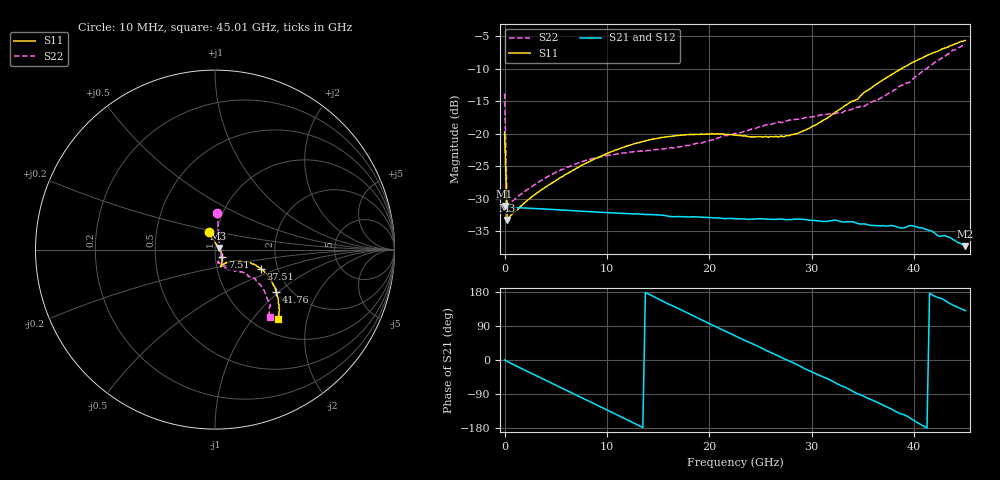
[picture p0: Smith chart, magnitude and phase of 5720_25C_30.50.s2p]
! Device:  ADRF5720
! Description: 0.5dB LSB GaAs MMIC 6-bit Digital Attenuator
! Frequency:  0.000009 -  40 GHz
! Ports:
!	RF1	= Port 1
!	RF2	= Port 2
! Vdd:  3.3 Volt
! Vss:  -3.3 Volt
! Control:  0/3.3 Volt
! State:  30.50 dB attenuation
! Data:  The device was measured using G-S-G Probes on a matrix board.
!  Data was collected using an calibrated 4 port network analyzer.
!  The reference plane for this measurement is at the launchers.
! Note:  Analog Devices supplies this data as a sample of measured data
!  for this product.  Your particular data for this product may vary.
!  Data was taken at 25 degrees C.
!  Analog Devices reserves the right to change this data at anytime.
# GHZ S DB R 45.0
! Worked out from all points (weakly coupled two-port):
!   181 points, 10 MHz to 45.01 GHz, reference 45 ohm
!   highest |S21| = -31.09 dB at 10 MHz (marker M1); lowest = -37.3 dB at 45.01 GHz (marker M2)
!   lowest |S11| = -33.2 dB at 260 MHz (marker M3), VSWR 1.04, Z = 46.8 + j0.872 ohm
!   |S11| at or under -10 dB: start of sweep to 38.74 GHz
!   |S22| runs from -31.3 to -6.2 dB; largest |S21 - S12| = 9.6e-05
!   S11 on the Smith chart (normalised r, x): 10 MHz: 0.92, +0.18; 7.51 GHz: 1.08, -0.09; 37.51 GHz: 1.63, -0.37; 41.76 GHz: 1.69, -0.97; 45.01 GHz: 1.27, -1.35
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0.01  -19.73 109.2  -31.09 0.2  -31.08 0.1  -13.80 86.3
0.26  -33.25 25.4  -31.29 -3.7  -31.29 -3.7  -31.32 17.3
0.51  -32.73 14.0  -31.30 -7.1  -31.31 -7.1  -30.64 7.1
3.26  -29.00 -18.9  -31.52 -43.6  -31.52 -43.6  -27.48 -34.1
7.51  -24.89 -46.2  -31.91 -99.1  -31.90 -99.1  -24.33 -65.8
7.76  -24.68 -47.3  -31.93 -102.4  -31.93 -102.4  -24.19 -67.1
11.51  -22.13 -59.8  -32.25 -151.6  -32.25 -151.6  -22.97 -76.4
15.26  -20.59 -67.7  -32.52 157.9  -32.52 157.9  -22.36 -76.1
20.26  -19.97 -71.3  -32.92 92.4  -32.93 92.5  -20.94 -66.3
22.76  -20.26 -69.2  -33.09 60.7  -33.09 60.7  -19.95 -62.3
27.26  -20.47 -51.6  -33.17 3.6  -33.17 3.6  -18.23 -58.6
30.26  -18.75 -33.7  -33.33 -34.2  -33.33 -34.2  -17.33 -56.7
34.51  -14.68 -20.6  -33.82 -89.3  -33.82 -89.2  -15.98 -47.8
35.01  -13.79 -20.2  -33.86 -94.7  -33.86 -94.7  -15.85 -46.4
37.51  -11.20 -22.6  -34.17 -125.8  -34.17 -125.6  -13.78 -38.9
37.76  -10.92 -23.2  -34.09 -129.3  -34.08 -129.2  -13.64 -38.5
38.76  -9.98 -25.3  -34.50 -142.5  -34.47 -142.3  -12.56 -38.3
39.76  -9.10 -28.5  -34.12 -155.8  -34.14 -155.7  -11.74 -36.6
41.76  -7.61 -34.8  -34.99 172.1  -34.99 172.1  -9.36 -39.1
42.26  -7.34 -36.4  -35.60 165.4  -35.63 165.3  -8.84 -40.1
43.76  -6.37 -42.1  -36.23 145.3  -36.23 145.3  -7.11 -45.3
45.01  -5.65 -47.9  -37.29 130.3  -37.27 130.6  -6.23 -50.8
